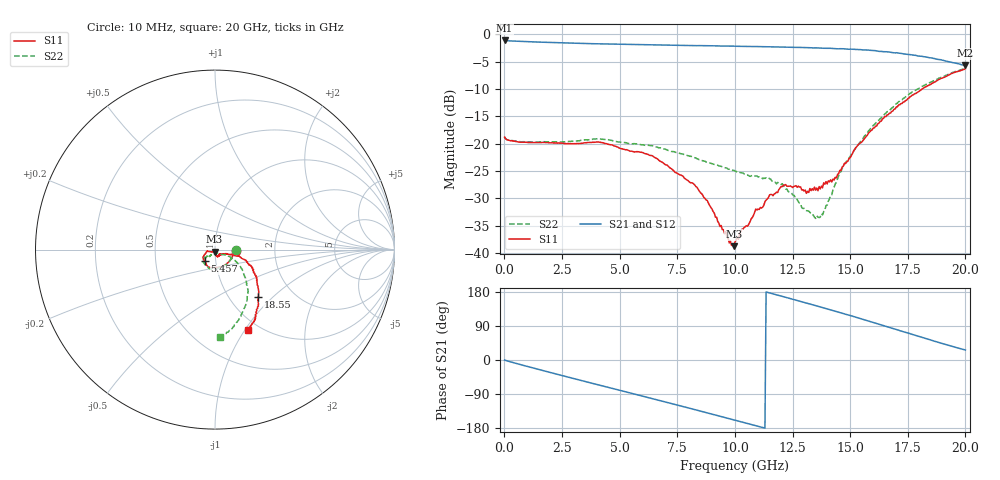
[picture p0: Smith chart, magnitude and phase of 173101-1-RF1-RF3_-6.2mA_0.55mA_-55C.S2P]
!  2-Port S-parameters saved by WinCal
! VAR MeasName=S-Parameters (CALIBRATED_DATA) read from VNA (N5242A)
! VAR MeasDate=2017-7-20 10:25:33
! VAR NAME=173101-1-RF1-RF3_-6.2mA_0.55mA_-55C
! VAR FILENAME=173101-1-RF1-RF3_-6.2mA_0.55mA_-55C.S2P
! VAR DATE=2017-7-20 10:25:33
! VAR PHYS_PORTS=1,2
# Hz S DB R 50
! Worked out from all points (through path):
!   401 points, 10 MHz to 20 GHz, reference 50 ohm
!   highest |S21| = -1.10 dB at 10 MHz (marker M1); lowest = -5.7 dB at 20 GHz (marker M2)
!   group delay of S21, straight-line fit = 45.8 ps
!   lowest |S11| = -38.7 dB at 9.955 GHz (marker M3), VSWR 1.02, Z = 49.7 - j1.12 ohm
!   |S11| at or under -10 dB: start of sweep to 18.12 GHz
!   |S22| runs from -33.7 to -6.2 dB; largest |S21 - S12| = 0.0091
!   S11 on the Smith chart (normalised r, x): 10 MHz: 1.26, -0.01; 5.457 GHz: 0.89, -0.11; 18.55 GHz: 1.36, -0.81; 20 GHz: 0.88, -1.03
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1e7  -18.79 -2.5  -1.10 -0.1  -1.11 -0.2  -18.74 -2.4
1.6092e9  -19.76 -53.3  -1.41 -26.9  -1.43 -26.9  -19.63 -51.3
3.358325e9  -19.91 -95.5  -1.64 -54.5  -1.65 -54.5  -19.35 -89.9
4.157925e9  -19.73 -111.9  -1.73 -66.9  -1.74 -66.9  -19.11 -105.3
5.457275e9  -21.35 -131.5  -1.83 -87.0  -1.84 -87.0  -19.95 -119.9
6.70665e9  -23.04 -150.8  -1.93 -106.5  -1.93 -106.5  -20.74 -134.4
8.30585e9  -27.81 -167.2  -2.05 -131.5  -2.06 -131.5  -22.60 -143.4
8.90555e9  -31.30 -155.0  -2.08 -141.1  -2.09 -141.0  -23.49 -139.4
9.755125e9  -38.12 -114.1  -2.13 -154.7  -2.14 -154.7  -24.66 -140.6
9.955025e9  -38.73 -103.7  -2.14 -157.9  -2.17 -157.9  -24.86 -140.7
1.0005e10  -37.97 -105.9  -2.16 -158.7  -2.18 -158.7  -24.98 -140.7
1.090455e10  -31.93 -78.6  -2.22 -173.1  -2.24 -173.2  -25.89 -131.3
1.205398e10  -27.83 -72.9  -2.32 168.0  -2.33 168.0  -27.30 -126.7
1.335332e10  -28.22 -50.5  -2.45 146.1  -2.42 146.0  -32.77 -86.3
1.36032e10  -28.58 -41.6  -2.46 141.8  -2.47 141.6  -33.42 -77.5
1.38031e10  -28.04 -41.7  -2.52 138.3  -2.51 138.2  -33.02 -68.7
1.430285e10  -26.63 -29.8  -2.58 129.6  -2.60 129.6  -27.98 -37.9
1.48026e10  -23.57 -21.0  -2.66 120.6  -2.67 120.7  -23.45 -27.1
1.585208e10  -17.82 -15.7  -2.90 101.6  -2.91 101.6  -17.42 -29.4
1.670165e10  -14.40 -20.5  -3.22 86.0  -3.30 85.5  -13.84 -39.0
1.855072e10  -8.96 -47.2  -4.30 51.6  -4.41 51.7  -8.63 -64.4
2e10  -6.28 -67.8  -5.68 26.4  -5.74 27.0  -6.19 -86.5
